(* Logix 5000 Routine export VSM_Program; software revision 20.01 *)

TYPE VSM_Config :
STRUCT
   Channel : Channel_Config[8];
   Number_of_Channels : INT;
   Switch_Hysteresis_Timer : INT;
END_STRUCT
END_TYPE

TYPE Communication_Status :
STRUCT
   Count : INT; {access Read Only}
   Status : INT; {access Read Only}
END_STRUCT
END_TYPE

TYPE Control_Bits :
STRUCT
   Switch_1_Control : BOOL;
   Switch_2_Control : BOOL;
   Reserved3 : BOOL;
   Reserved4 : BOOL;
   Reserved5 : BOOL;
   Switch_1_Enabled : BOOL;
   Switch_1_Failsafe : BOOL;
   Switch_1_Latching : BOOL;
   Bad_Sensor_Switch_Select : BOOL;
   Switch_2_Enable : BOOL;
   Switch_2_Failsafe : BOOL;
   Switch_2_Latching : BOOL;
   Reserved13 : BOOL;
   Reserved14 : BOOL;
   Reserved15 : BOOL;
   Startup_Lockout : BOOL;
END_STRUCT
END_TYPE

TYPE Key_Command :
STRUCT
   Command : SINT;
   Compliment : SINT;
   Arg_1 : SINT;
   Arg_2 : SINT;
END_STRUCT
END_TYPE

TYPE VSM_Output :
STRUCT
   Channel_Gain : INT[8];
   Lag_Filter : INT;
   Status_Control : INT;
   Control_Bits : Control_Bits;
END_STRUCT
END_TYPE

TYPE Diagnostic_Bits :
STRUCT
   Reserved1 : BOOL; {access Read Only}
   Reserved2 : BOOL; {access Read Only}
   SW1_Active : BOOL; {access Read Only}
   SW2_Active : BOOL; {access Read Only}
   Reserved5 : BOOL; {access Read Only}
   Reserved6 : BOOL; {access Read Only}
   Reserved7 : BOOL; {access Read Only}
   Reserved8 : BOOL; {access Read Only}
   CAL_R_W : BOOL; {access Read Only}
   Watchdog : BOOL; {access Read Only}
   Reset : BOOL; {access Read Only}
   Reserved12 : BOOL; {access Read Only}
   Startup_Locked_Out : BOOL; {access Read Only}
   Alarm : BOOL; {access Read Only}
   Reserved15 : BOOL; {access Read Only}
   Reserved16 : BOOL; {access Read Only}
END_STRUCT
END_TYPE

TYPE Channel_Config :
STRUCT
   Reserved : INT;
   Alarm_Setpoint : INT;
   Shutdown_Setpoint : INT;
   Bad_Sensor_Setpoint : INT;
   Start_Delay : INT;
   Trip_Delay : INT;
END_STRUCT
END_TYPE

TYPE VSM_Input :
STRUCT
   Vibration : INT[8]; {access Read Only}
   Spply_Voltage : REAL; {access Read Only}
   Diagnostics : Diagnostic_Bits; {access Read Only}
   Bad_Sensor_Bits : SINT; {access Read Only}
   Critical_High_Bits : SINT; {access Read Only}
   High_Vibration_Bits : SINT; {access Read Only}
   Channel_Armed_Bits : SINT; {access Read Only}
   Communication_Status : Communication_Status; {access Read Only}
   Control_Bits_Echo : Control_Bits; {access Read Only}
END_STRUCT
END_TYPE

VAR_GLOBAL   (* controller tags *)
   VSM_Load_Defaults : BOOL;
   VSM_Keycommand_Message : MESSAGE;
        MessageParameters(MessageType := CIP Generic, RequestedLength := 4, ConnectedFlag := 2, ConnectionPath := VSMPlus, ServiceCode := 16#004b, ObjectType := 16#0069, TargetObject := 1, LocalElement := VSM_Keycommand)
   VSM_Reconfigure : BOOL;
   VSM_Reconfigure_Message : MESSAGE;
        MessageParameters(MessageType := Module Reconfigure, RequestedLength := 1, ConnectionPath := VSMPlus)
   asint : SINT := 71;
   VSM_Control_Reset_Trigger : BOOL;
   VSM_Clear_Alarms_Trigger : BOOL;
   VSM_Input : VSM_Input := (Vibration[0] := 899, Vibration[1] := 28, Vibration[2] := 28, Vibration[3] := 28, Vibration[4] := 28, Vibration[5] := 28, Vibration[6] := 28, Vibration[7] := 28, Spply_Voltage := 22.79, Channel_Armed_Bits := -1, Control_Bits_Echo.Switch_1_Failsafe := 1);
   VSM_Config : VSM_Config := (Channel[0].Alarm_Setpoint := 999, Channel[0].Shutdown_Setpoint := 999, Channel[1].Alarm_Setpoint := 999, Channel[1].Shutdown_Setpoint := 999, Channel[2].Alarm_Setpoint := 999, Channel[2].Shutdown_Setpoint := 999, Channel[3].Alarm_Setpoint := 999, Channel[3].Shutdown_Setpoint := 999, Channel[4].Alarm_Setpoint := 999, Channel[4].Shutdown_Setpoint := 999, Channel[5].Alarm_Setpoint := 999, Channel[5].Shutdown_Setpoint := 999, Channel[6].Alarm_Setpoint := 999, Channel[6].Shutdown_Setpoint := 999, Channel[7].Alarm_Setpoint := 999, Channel[7].Shutdown_Setpoint := 999, Number_of_Channels := 8);
   VSM_Clear_Timers_Trigger : BOOL;
   VSM_Loop_Counter : SINT := 8;
   VSM_Keycommand : Key_Command := (Command := 6, Compliment := -7);
   VSM_Output : VSM_Output := (Channel_Gain[0] := 14, Channel_Gain[1] := 14, Channel_Gain[2] := 14, Channel_Gain[3] := 14, Channel_Gain[4] := 14, Channel_Gain[5] := 14, Channel_Gain[6] := 14, Channel_Gain[7] := 14, Lag_Filter := 240, Control_Bits.Switch_1_Failsafe := 1);
END_VAR

PROGRAM MainProgram

ROUTINE VSM_Program   (* ladder *)
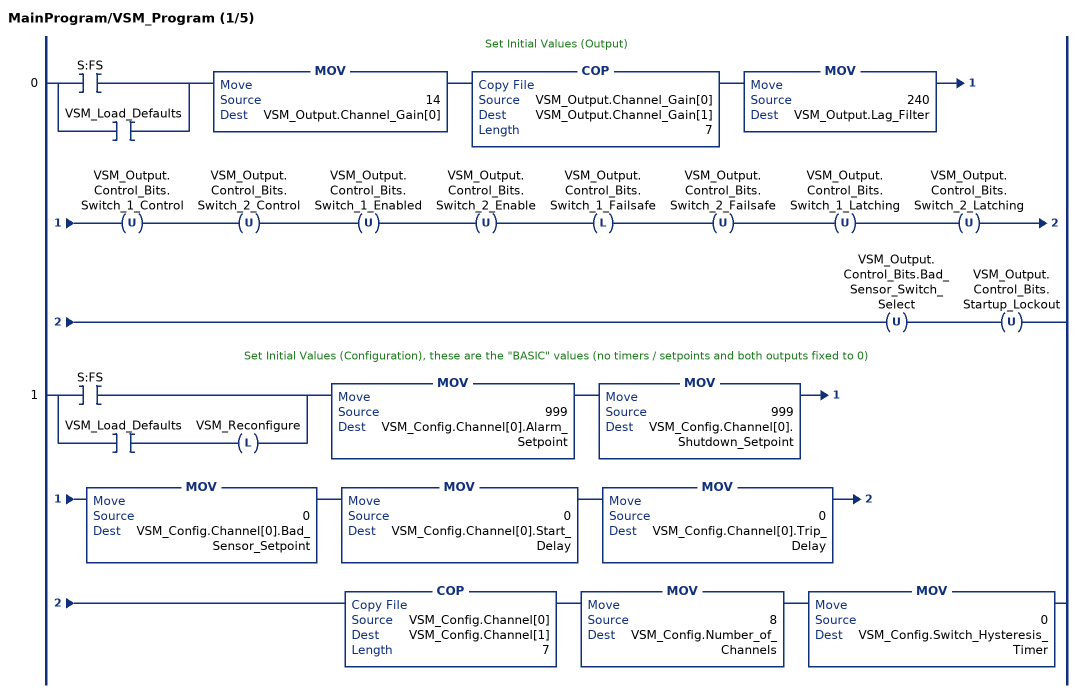
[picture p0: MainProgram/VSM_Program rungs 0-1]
   // Set Initial Values (Output)
   0: [XIC(S:FS) ,XIC(VSM_Load_Defaults) ]MOV(14,VSM_Output.Channel_Gain[0])COP(VSM_Output.Channel_Gain[0],VSM_Output.Channel_Gain[1],7)MOV(240,VSM_Output.Lag_Filter)OTU(VSM_Output.Control_Bits.Switch_1_Control)OTU(VSM_Output.Control_Bits.Switch_2_Control)OTU(VSM_Output.Control_Bits.Switch_1_Enabled)OTU(VSM_Output.Control_Bits.Switch_2_Enable)OTL(VSM_Output.Control_Bits.Switch_1_Failsafe)OTU(VSM_Output.Control_Bits.Switch_2_Failsafe)OTU(VSM_Output.Control_Bits.Switch_1_Latching)OTU(VSM_Output.Control_Bits.Switch_2_Latching)OTU(VSM_Output.Control_Bits.Bad_Sensor_Switch_Select)OTU(VSM_Output.Control_Bits.Startup_Lockout);
   // Set Initial Values (Configuration), these are the "BASIC" values (no timers / setpoints and both outputs fixed to 0)
   1: [XIC(S:FS) ,XIC(VSM_Load_Defaults) OTL(VSM_Reconfigure) ]MOV(999,VSM_Config.Channel[0].Alarm_Setpoint)MOV(999,VSM_Config.Channel[0].Shutdown_Setpoint)MOV(0,VSM_Config.Channel[0].Bad_Sensor_Setpoint)MOV(0,VSM_Config.Channel[0].Start_Delay)MOV(0,VSM_Config.Channel[0].Trip_Delay)COP(VSM_Config.Channel[0],VSM_Config.Channel[1],7)MOV(8,VSM_Config.Number_of_Channels)MOV(0,VSM_Config.Switch_Hysteresis_Timer);
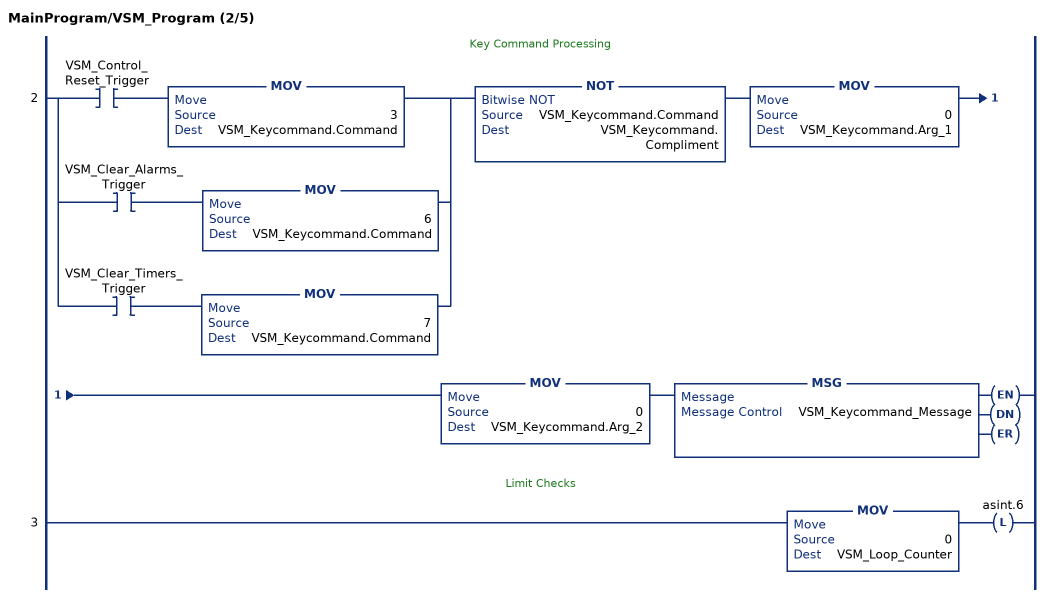
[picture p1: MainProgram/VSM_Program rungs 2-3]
   // Key Command Processing
   2: [XIC(VSM_Control_Reset_Trigger) MOV(3,VSM_Keycommand.Command) ,XIC(VSM_Clear_Alarms_Trigger) MOV(6,VSM_Keycommand.Command) ,XIC(VSM_Clear_Timers_Trigger) MOV(7,VSM_Keycommand.Command) ]NOT(VSM_Keycommand.Command,VSM_Keycommand.Compliment)MOV(0,VSM_Keycommand.Arg_1)MOV(0,VSM_Keycommand.Arg_2)MSG(VSM_Keycommand_Message);
   // Limit Checks
   3: MOV(0,VSM_Loop_Counter)OTL(asint.6);
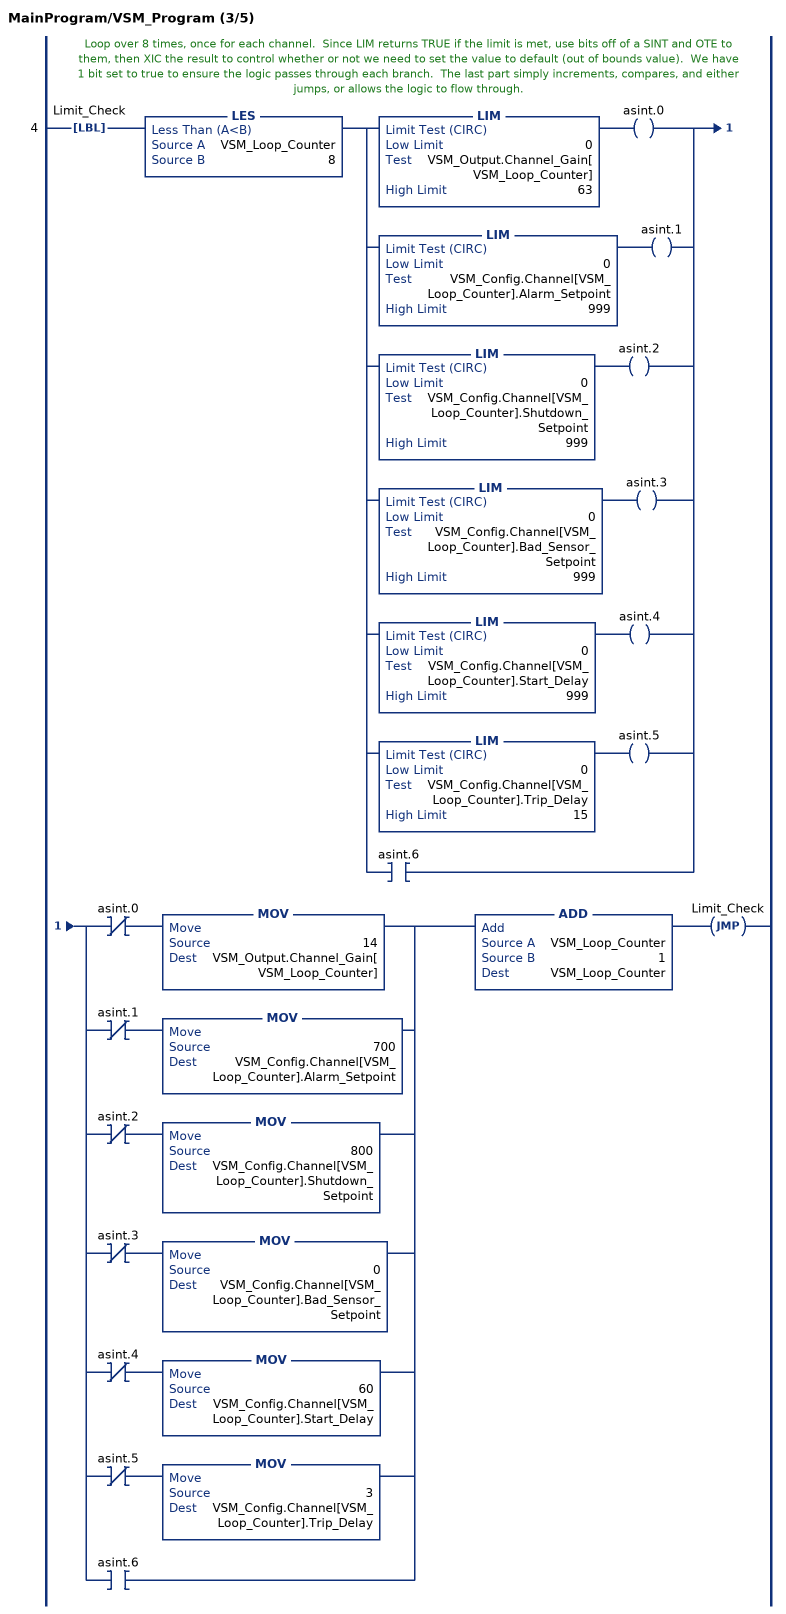
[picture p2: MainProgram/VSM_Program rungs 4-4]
   // Loop over 8 times, once for each channel.  Since LIM returns TRUE if the limit is met, use bits off of a SINT and OTE to them, then XIC the result to control whether or not we need to set the value to default (out of bounds value).  We have 1 bit set to true to ensure the logic passes through each branch.  The last part simply increments, compares, and either jumps, or allows the logic to flow through.
   4: LBL(Limit_Check)LES(VSM_Loop_Counter,8)[LIM(0,VSM_Output.Channel_Gain[VSM_Loop_Counter],63) OTE(asint.0) ,LIM(0,VSM_Config.Channel[VSM_Loop_Counter].Alarm_Setpoint,999) OTE(asint.1) ,LIM(0,VSM_Config.Channel[VSM_Loop_Counter].Shutdown_Setpoint,999) OTE(asint.2) ,LIM(0,VSM_Config.Channel[VSM_Loop_Counter].Bad_Sensor_Setpoint,999) OTE(asint.3) ,LIM(0,VSM_Config.Channel[VSM_Loop_Counter].Start_Delay,999) OTE(asint.4) ,LIM(0,VSM_Config.Channel[VSM_Loop_Counter].Trip_Delay,15) OTE(asint.5) ,XIC(asint.6) ][XIO(asint.0) MOV(14,VSM_Output.Channel_Gain[VSM_Loop_Counter]) ,XIO(asint.1) MOV(700,VSM_Config.Channel[VSM_Loop_Counter].Alarm_Setpoint) ,XIO(asint.2) MOV(800,VSM_Config.Channel[VSM_Loop_Counter].Shutdown_Setpoint) ,XIO(asint.3) MOV(0,VSM_Config.Channel[VSM_Loop_Counter].Bad_Sensor_Setpoint) ,XIO(asint.4) MOV(60,VSM_Config.Channel[VSM_Loop_Counter].Start_Delay) ,XIO(asint.5) MOV(3,VSM_Config.Channel[VSM_Loop_Counter].Trip_Delay) ,XIC(asint.6) ]ADD(VSM_Loop_Counter,1,VSM_Loop_Counter)JMP(Limit_Check);
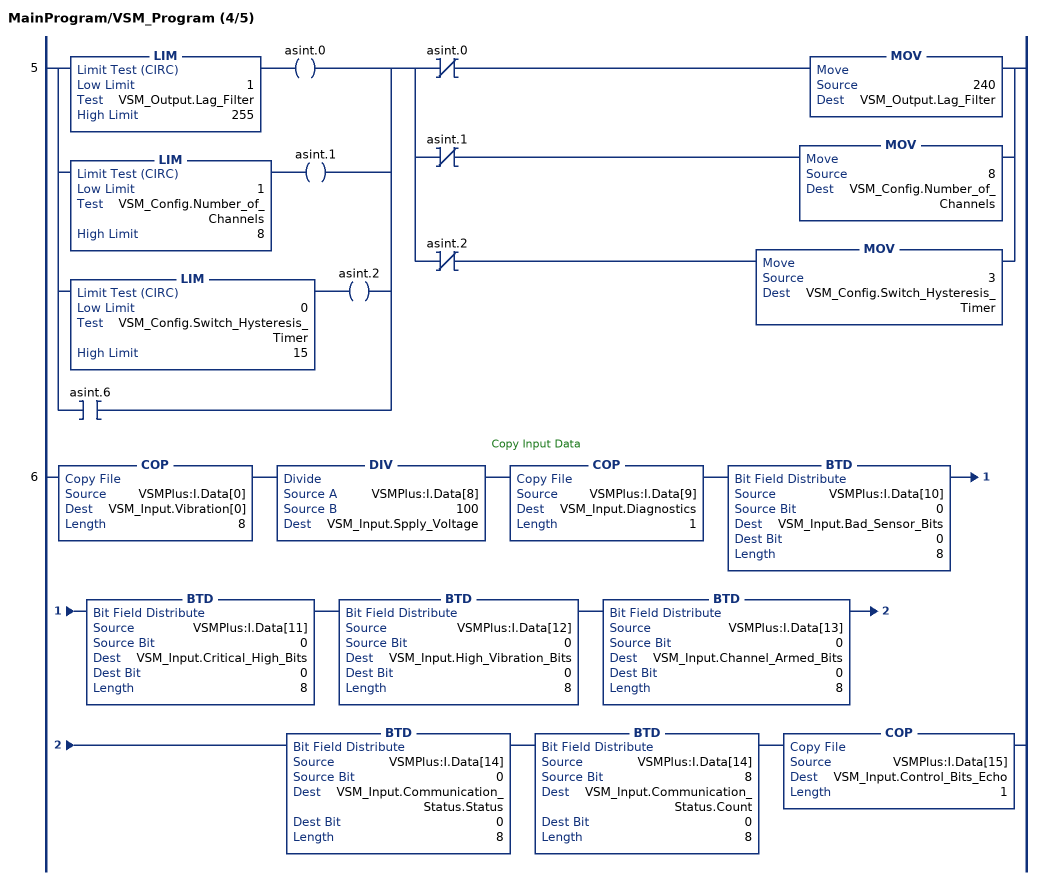
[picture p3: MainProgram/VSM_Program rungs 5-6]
   5: [LIM(1,VSM_Output.Lag_Filter,255) OTE(asint.0) ,LIM(1,VSM_Config.Number_of_Channels,8) OTE(asint.1) ,LIM(0,VSM_Config.Switch_Hysteresis_Timer,15) OTE(asint.2) ,XIC(asint.6) ][XIO(asint.0) MOV(240,VSM_Output.Lag_Filter) ,XIO(asint.1) MOV(8,VSM_Config.Number_of_Channels) ,XIO(asint.2) MOV(3,VSM_Config.Switch_Hysteresis_Timer) ];
   // Copy Input Data
   6: COP(VSMPlus:I.Data[0],VSM_Input.Vibration[0],8)DIV(VSMPlus:I.Data[8],100,VSM_Input.Spply_Voltage)COP(VSMPlus:I.Data[9],VSM_Input.Diagnostics,1)BTD(VSMPlus:I.Data[10],0,VSM_Input.Bad_Sensor_Bits,0,8)BTD(VSMPlus:I.Data[11],0,VSM_Input.Critical_High_Bits,0,8)BTD(VSMPlus:I.Data[12],0,VSM_Input.High_Vibration_Bits,0,8)BTD(VSMPlus:I.Data[13],0,VSM_Input.Channel_Armed_Bits,0,8)BTD(VSMPlus:I.Data[14],0,VSM_Input.Communication_Status.Status,0,8)BTD(VSMPlus:I.Data[14],8,VSM_Input.Communication_Status.Count,0,8)COP(VSMPlus:I.Data[15],VSM_Input.Control_Bits_Echo,1);
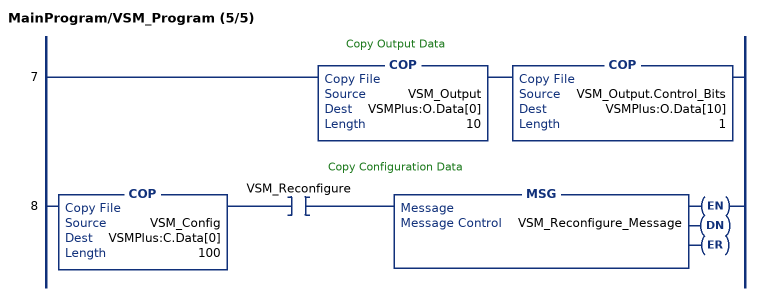
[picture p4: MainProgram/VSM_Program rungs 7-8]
   // Copy Output Data
   7: COP(VSM_Output,VSMPlus:O.Data[0],10)COP(VSM_Output.Control_Bits,VSMPlus:O.Data[10],1);
   // Copy Configuration Data
   8: COP(VSM_Config,VSMPlus:C.Data[0],100)XIC(VSM_Reconfigure)MSG(VSM_Reconfigure_Message);
END_ROUTINE
END_PROGRAM
